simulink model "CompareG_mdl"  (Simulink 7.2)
settings: Solver=ode45  StartTime=0.0  StopTime=100  RelTol=1e-3
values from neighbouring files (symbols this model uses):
  Ts = 0.1    [IdentificazioneG.m]
libraries: cstblocks x1

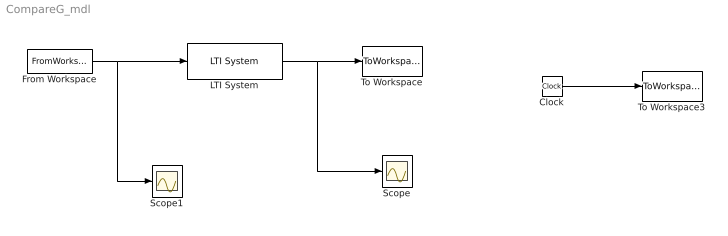
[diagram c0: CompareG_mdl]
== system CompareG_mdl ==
  Clock : Clock
  From Workspace : FromWorkspace  VariableName=[timed u]  SampleTime=0
  LTI System : cstblocks/LTI System  SystemSampleTime=-1  sys=Gi  IC=[]
  Scope : Scope
  Scope1 : Scope
  To Workspace : ToWorkspace  VariableName=yi  SampleTime=Ts  SaveFormat=Array
  To Workspace3 : ToWorkspace  VariableName=time  SampleTime=-1  SaveFormat=Array
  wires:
  From Workspace/1 -> LTI System/1, Scope1/1
  LTI System/1 -> To Workspace/1, Scope/1
  Clock/1 -> To Workspace3/1
